(* FB_Cylinder		- number of control signals控制信号数量:
							one direction is controllable一个方向是可控的
					- type of feedback signal反馈信号的类型:
							feedback in base and work position基准和工作位置的反馈		*)
						
FUNCTION_BLOCK FB_Cylinder //IMPLEMENTS I_Cylinder
VAR_INPUT
	bAtBasePos		AT %I*	: BOOL;		// Hardware input signal: cylinder is at base position硬件输入信号：气缸处于基准位置
	bAtWorkPos		AT %I*	: BOOL;		// Hardware input signal: cylinder is at work position硬件输入信号：气缸在工作位置
END_VAR
VAR_OUTPUT
	bMoveToWork		AT %Q*	: BOOL;		// Hardware output signal to move cylinder to work position将气缸移动到工作位置的硬件输出信号
END_VAR

// =========================================================
;
// =========================================================

PROPERTY PUBLIC bState_AtBasePos : BOOL
GET
bState_AtBasePos := bAtBasePos;
END_GET
END_PROPERTY

PROPERTY PUBLIC bState_AtWorkPos : BOOL
GET
bState_AtWorkPos := bAtWorkPos;
END_GET
END_PROPERTY

PROPERTY PUBLIC bState_MoveToWork : BOOL
GET
bState_MoveToWork := bMoveToWork;
END_GET
END_PROPERTY

METHOD MoveToBase
VAR_INPUT
END_VAR
// =========================================================
	
StateMachine(	bBasePosReq := TRUE,
				bWorkPosReq	:= FALSE );
							
// =========================================================
END_METHOD

METHOD MoveToWork
VAR_INPUT
END_VAR
// =========================================================
	
StateMachine(	bBasePosReq := FALSE,
				bWorkPosReq	:= TRUE );
								
// =========================================================
END_METHOD

METHOD Reset
VAR_INPUT
END_VAR
// =========================================================

bMoveToWork := FALSE;

// =========================================================
END_METHOD

METHOD PROTECTED StateMachine
VAR_INPUT
	bBasePosReq		: BOOL;
	bWorkPosReq		: BOOL;
END_VAR
// =========================================================
// Base or work position requested被要求移动至基准或工作位置
		
	IF bWorkPosReq THEN
		bMoveToWork := TRUE;
	END_IF
	
	IF bBasePosReq OR NOT bWorkPosReq THEN
		bMoveToWork := FALSE;
	END_IF

// =========================================================
END_METHOD

END_FUNCTION_BLOCK
